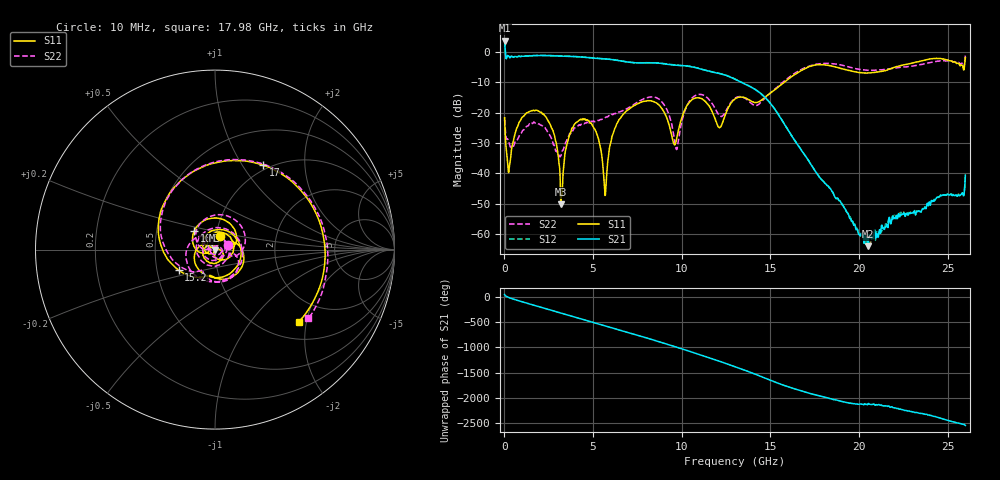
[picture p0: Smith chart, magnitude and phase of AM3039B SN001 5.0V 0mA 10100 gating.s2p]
!Agilent Technologies,E8364B,MY43040894,A.07.50.67
!Agilent E8364B: A.07.50.67
!Date: Tuesday, June 28, 2016 08:09:04
!Correction: S11(Full 2 Port(1,2))
!S21(Full 2 Port(1,2))
!S12(Full 2 Port(1,2))
!S22(Full 2 Port(1,2))
!S2P File: Measurements: S11, S21, S12, S22:
# Hz S  dB  R 50
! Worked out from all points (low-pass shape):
!   1601 points, 10 MHz to 26 GHz, reference 50 ohm
!   highest |S21| = 3.72 dB at 10 MHz (marker M1); lowest = -64.0 dB at 20.51 GHz (marker M2)
!   |S21| within 3 dB of the highest: start of sweep to 44.03 MHz
!   lowest |S11| = -50.2 dB at 3.178 GHz (marker M3), VSWR 1.01, Z = 50 - j0.308 ohm
!   |S11| at or under -10 dB: start of sweep to 15.77 GHz
!   |S22| runs from -34.6 to -1.0 dB; largest |S21 - S12| = 0.026
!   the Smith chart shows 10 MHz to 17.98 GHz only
!   S11 on the Smith chart (normalised r, x): 10 MHz: 1.05, +0.16; 10.5 GHz: 0.78, +0.17; 15.2 GHz: 0.65, -0.16; 17 GHz: 0.94, +1.25; 17.98 GHz: 1.38, -1.80
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1e7  -21.68 69.6  3.72 40.9  3.79 41.7  -22.30 18.0
7.409688e8  -24.60 131.2  -1.60 -75.0  -1.55 -74.8  -28.78 169.4
1.731838e9  -19.36 30.9  -1.23 -177.0  -1.19 -176.7  -23.43 22.0
3.177531e9  -50.19 -94.6  -1.35 37.6  -1.28 37.8  -34.25 92.0
4.347081e9  -22.30 -101.7  -1.68 -80.9  -1.64 -80.8  -23.74 -128.6
5.679069e9  -47.32 9.3  -2.31 142.9  -2.26 143.1  -21.63 -21.7
6.101406e9  -27.31 -150.7  -2.55 99.0  -2.48 99.1  -20.66 -103.9
7.141006e9  -18.32 62.8  -3.47 -7.1  -3.43 -7.0  -17.91 69.1
8.684162e9  -17.29 -142.1  -3.68 -167.9  -3.62 -167.7  -15.43 -161.0
9.707519e9  -28.74 -162.8  -4.39 81.4  -4.34 81.4  -32.16 143.0
1.050346e10  -16.14 137.6  -4.80 -8.5  -4.76 -8.5  -15.70 122.4
1.188418e10  -22.14 1.5  -6.80 -167.4  -6.74 -167.5  -18.61 -17.5
1.3005e10  -15.49 -16.5  -8.99 54.3  -8.95 54.1  -15.21 -46.9
1.519791e10  -12.68 -150.3  -18.44 120.2  -18.37 120.1  -12.54 -163.8
1.700096e10  -5.32 60.1  -34.50 -89.5  -34.46 -89.7  -5.07 54.0
1.734208e10  -4.55 25.1  -37.58 -124.3  -37.53 -124.3  -4.38 22.5
1.797559e10  -4.21 -40.9  -42.50 -178.9  -42.58 -178.7  -3.78 -36.4
2.050961e10  -6.95 105.2  -64.01 39.0  -63.55 24.8  -6.04 115.6
2.167916e10  -5.71 24.5  -55.29 -1.5  -55.21 -10.9  -5.57 31.8
2.322232e10  -3.34 -92.3  -53.07 -127.3  -52.75 -131.7  -4.46 -81.1
2.432689e10  -2.13 177.9  -48.45 146.2  -48.53 145.2  -3.10 -165.5
2.6e10  -1.82 -13.1  -40.60 -25.9  -40.41 -25.3  -0.97 19.2
